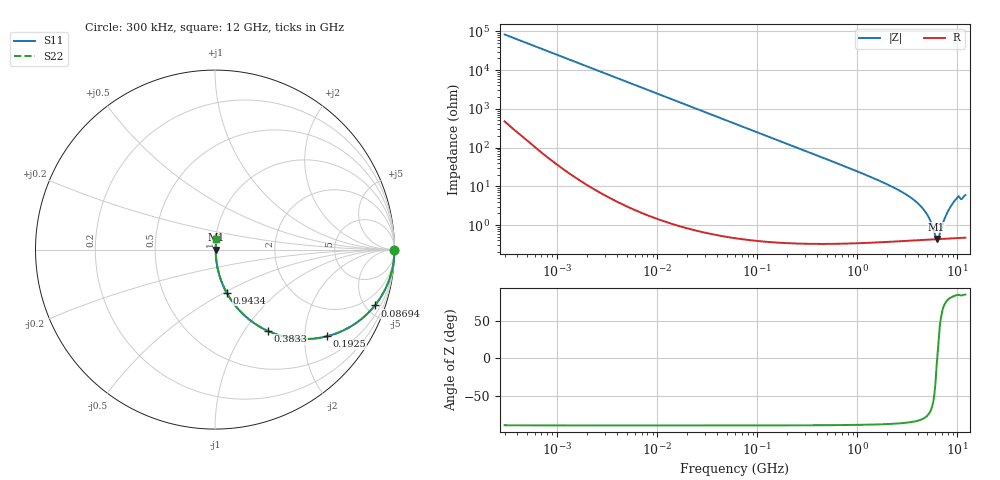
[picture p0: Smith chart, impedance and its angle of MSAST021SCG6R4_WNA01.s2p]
! MSAST021SCG6R4_WNA01  S-PARAMETER MODEL  ( General Type )
! Model Generated by TAIYO YUDEN Corporation (http://www.ty-top.com)
! Version 2.0
! TAIYO YUDEN Control No. 181101
! Copyright(c) 2015 TAIYO YUDEN CO.,LTD. All Rights Reserved.
! Product Description (link to TY-COMPAS)
! https://ds.yuden.co.jp/TYCOMPAS/or/detail?pn=MSAST021SCG6R4CWNA01&u=M
! Products Name : Multilayer Ceramic Capacitors
! Characteristics :
!  Capacitance : 6.4 pF , Rated Voltage : 25V , TCC : CG / C0G
!  Case Size : 0.25 x 0.125 / 0.0098 x 0.0049 [mm/inch] , Thickness : 0.125 / 0.0049 [mm/inch]
!  (Conditions: Temperature = 25 degC , DC Bias Current/Voltage = 0A / 0V)
! External Node Assignments :
!  1  o---| |---o  2
! GND o---------o GND
! Frequency Range : 0.3MHz  -  12000MHz  [ 401 STEP ]
# MHz S RI R 50
! Freq[MHz].  S11 Real  S11 Imag  S21 Real  S21 Imag  S12 Real  S12 Imag  S22 Real  S22 Imag
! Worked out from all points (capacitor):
!   401 points, 300 kHz to 12 GHz, reference 50 ohm
!   read as one part in series: C = 6.4 pF near 316.3 kHz
!   lowest |Z| = 439 mohm at 6.188 GHz (marker M1)
!   series resonance near 6.274 GHz, so ESL is about 100 pH
!   S11 on the Smith chart (normalised r, x): 300 kHz: open; 86.94 MHz: 1.01, -5.72; 192.5 MHz: 1.01, -2.58; 383.3 MHz: 1.01, -1.29; 943.4 MHz: 1.01, -0.52; 12 GHz: 1.01, +0.12
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0.3  1 -0.00121  8.34e-06 0.00121  8.34e-06 0.00121  1 -0.00121
1.769972  0.9999 -0.00712  5.73e-05 0.00712  5.73e-05 0.00712  0.9999 -0.00712
10.44266  0.9982 -0.0419  0.00178 0.0419  0.00178 0.0419  0.9982 -0.0419
27.10171  0.9882 -0.1077  0.0118 0.1077  0.0118 0.1077  0.9882 -0.1077
60  0.9448 -0.2279  0.0552 0.2279  0.0552 0.2279  0.9448 -0.2279
86.94074  0.8907 -0.3113  0.1093 0.3113  0.1093 0.3113  0.8907 -0.3113
129.3602  0.7864 -0.4089  0.2136 0.4089  0.2136 0.4089  0.7864 -0.4089
192.4766  0.6246 -0.4829  0.3754 0.4829  0.3754 0.4829  0.6246 -0.4829
353.9943  0.3298 -0.4678  0.6702 0.4678  0.6702 0.4678  0.3298 -0.4678
383.2761  0.2956 -0.4538  0.7044 0.4538  0.7044 0.4538  0.2956 -0.4538
585.5907  0.1525 -0.3556  0.8475 0.3556  0.8475 0.3556  0.1525 -0.3556
943.3804  0.065 -0.24  0.935 0.24  0.935 0.24  0.065 -0.24
2088.533  0.0146 -0.1038  0.9854 0.1038  0.9854 0.1038  0.0146 -0.1038
3190.978  0.00718 -0.057  0.9928 0.057  0.9928 0.057  0.00718 -0.057
4270.516  0.00503 -0.0308  0.995 0.0308  0.995 0.0308  0.00503 -0.0308
5140.631  0.00443 -0.0155  0.9956 0.0155  0.9956 0.0155  0.00443 -0.0155
6188.031  0.0043 -0.000753  0.9957 0.000753  0.9957 0.000753  0.0043 -0.000753
6524.734  0.00434 0.00238  0.9957 -0.00238  0.9957 -0.00238  0.00434 0.00238
7648.807  0.00471 0.0165  0.9953 -0.0165  0.9953 -0.0165  0.00471 0.0165
8966.534  0.00578 0.0353  0.9942 -0.0353  0.9942 -0.0353  0.00578 0.0353
9968.853  0.00716 0.0505  0.9928 -0.0505  0.9928 -0.0505  0.00716 0.0505
12000  0.00815 0.0585  0.9918 -0.0585  0.9918 -0.0585  0.00815 0.0585
